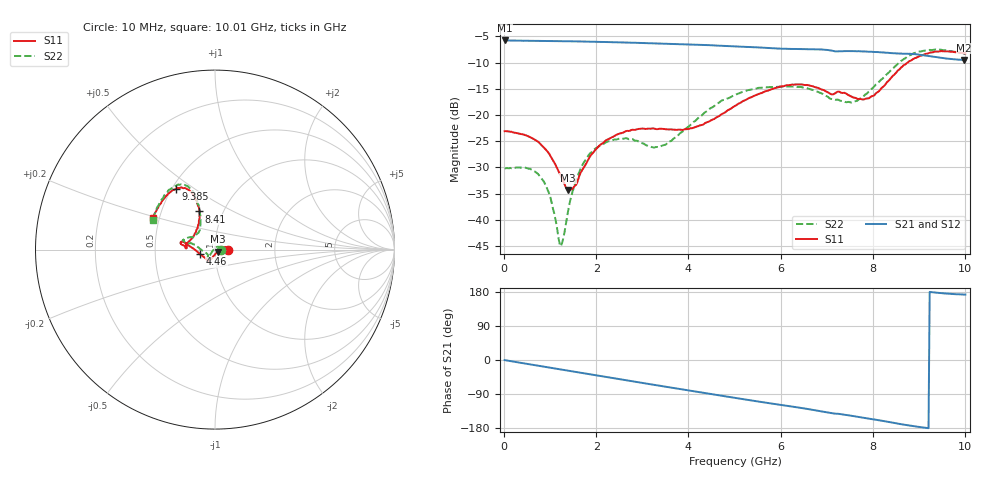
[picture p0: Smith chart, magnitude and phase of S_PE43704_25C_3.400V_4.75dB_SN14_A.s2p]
! Device ID: PE43704
! Dir: z:\PE43704\PE43704_Char_1_20130516\PE43704\AMB\3p400V\4p75dB
! Serial: 14
! Insertion: A
! Impedance: 50 ohm
! Temp: Amb
! VDD: 3.400V
! Attenuation Step: 4.75dB
! IDD: 1.140926e-01mA
#  Hz  S  RI  R  50
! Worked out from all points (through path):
!   401 points, 10 MHz to 10.01 GHz, reference 50 ohm
!   highest |S21| = -5.78 dB at 10 MHz (marker M1); lowest = -9.5 dB at 9.985 GHz (marker M2)
!   group delay of S21, straight-line fit = 53.5 ps
!   lowest |S11| = -34.3 dB at 1.385 GHz (marker M3), VSWR 1.04, Z = 51.6 - j1.13 ohm
!   |S11| at or under -10 dB: start of sweep to 8.757 GHz
!   |S22| runs from -45.0 to -7.5 dB; largest |S21 - S12| = 0.0038
!   S11 on the Smith chart (normalised r, x): 10 MHz: 1.15, +0.00; 4.46 GHz: 0.84, -0.04; 8.41 GHz: 0.77, +0.35; 9.385 GHz: 0.52, +0.42; 10.01 GHz: 0.46, +0.19
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1e7  0.0701 0.000149  0.5142 -0.00198  0.5143 -0.00189  0.0309 0.000357
5.1e8  0.0613 0.0142  0.5019 -0.0931  0.5017 -0.093  0.025 0.0182
8.1e8  0.0496 0.0143  0.4874 -0.1454  0.4874 -0.1453  0.0161 0.0188
9.85e8  0.0409 0.00992  0.477 -0.1747  0.4769 -0.1746  0.00879 0.0151
1.235e9  0.0258 -0.00212  0.4581 -0.216  0.4582 -0.2158  -0.00371 0.00419
1.385e9  0.0158 -0.0109  0.4448 -0.2393  0.4449 -0.2392  -0.0112 -0.00416
1.685e9  -0.00136 -0.0293  0.4149 -0.2838  0.415 -0.2836  -0.0235 -0.0225
1.96e9  -0.0139 -0.0431  0.3831 -0.3205  0.3833 -0.3203  -0.0306 -0.0357
2.36e9  -0.0255 -0.0563  0.3317 -0.3671  0.3319 -0.367  -0.0372 -0.0439
3.36e9  -0.0393 -0.0624  0.1827 -0.4451  0.1832 -0.4449  -0.0423 -0.0254
4.46e9  -0.0836 -0.0249  0.00465 -0.4636  0.00499 -0.4639  -0.1114 0.0265
5.01e9  -0.1217 0.00604  -0.0778 -0.4439  -0.0775 -0.4443  -0.1511 0.0353
5.985e9  -0.1809 0.0447  -0.2017 -0.3797  -0.1998 -0.3804  -0.1794 0.0509
6.685e9  -0.1865 0.0286  -0.2802 -0.3185  -0.2803 -0.3179  -0.1624 0.0624
7.585e9  -0.1361 0.0539  -0.3461 -0.2143  -0.3456 -0.2138  -0.0889 0.1007
7.96e9  -0.1044 0.1072  -0.3652 -0.1657  -0.3654 -0.1665  -0.0814 0.1553
8.36e9  -0.0861 0.1981  -0.3748 -0.1091  -0.3748 -0.1107  -0.0904 0.2416
8.41e9  -0.0878 0.2124  -0.3754 -0.1019  -0.3753 -0.103  -0.096 0.2542
8.86e9  -0.1273 0.3133  -0.3797 -0.0389  -0.3771 -0.0405  -0.1503 0.3517
9.385e9  -0.2177 0.3387  -0.3556 0.0146  -0.3564 0.0157  -0.2394 0.3438
9.985e9  -0.3386 0.1881  -0.3317 0.0428  -0.3331 0.0439  -0.3409 0.1765
1.001e10  -0.3445 0.1775  -0.3324 0.0429  -0.3349 0.0434  -0.3448 0.1675
